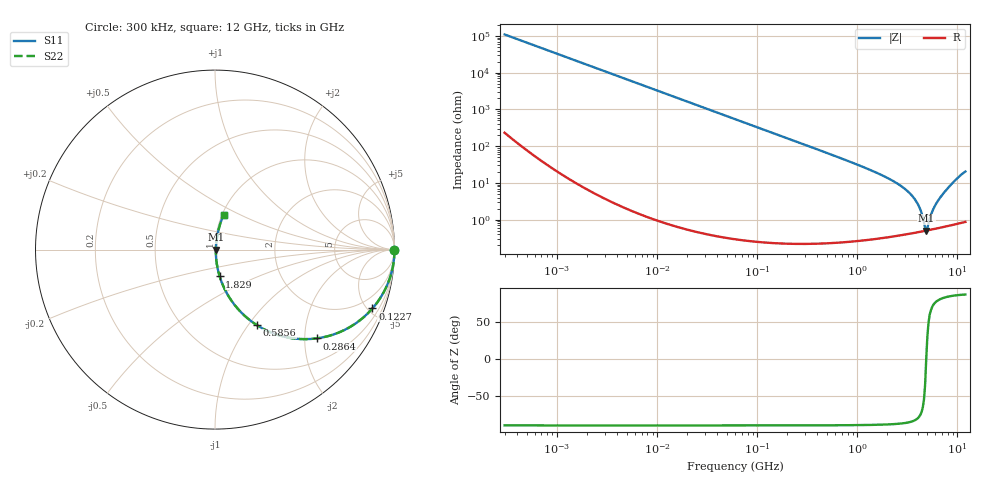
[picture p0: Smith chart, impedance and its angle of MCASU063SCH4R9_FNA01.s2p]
! MCASU063SCH4R9_FNA01  S-PARAMETER MODEL  ( General Type )
! Model Generated by TAIYO YUDEN Corporation (http://www.ty-top.com)
! Version 1.0
! TAIYO YUDEN Control No. 130801
! Copyright(c) 2013 TAIYO YUDEN CO.,LTD. All Rights Reserved.
! Product Description (link to TY-COMPAS)
! https://ds.yuden.co.jp/TYCOMPAS/or/detail?pn=MCASU063SCH4R9CFNA01&u=M
! Products Name : Multilayer Ceramic Capacitors
! Characteristics :
!  Capacitance : 4.9 pF , Rated Voltage : 50V , TCC : CH / C0H
!  Case Size : 0.6 x 0.3 / 0.024 x 0.012 [mm/inch] , Thickness : 0.3 / 0.012 [mm/inch]
!  (Conditions: Temperature = 25 degC , DC Bias Current/Voltage = 0A / 0V)
! External Node Assignments :
!  1  o---| |---o  2
! GND o---------o GND
! Frequency Range : 0.3MHz  -  12000MHz  [ 401 STEP ]
# MHz S RI R 50
! Freq[MHz].  S11 Real  S11 Imag  S21 Real  S21 Imag  S12 Real  S12 Imag  S22 Real  S22 Imag
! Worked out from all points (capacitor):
!   401 points, 300 kHz to 12 GHz, reference 50 ohm
!   read as one part in series: C = 4.85 pF near 316.3 kHz
!   lowest |Z| = 503 mohm at 4.875 GHz (marker M1)
!   series resonance near 4.876 GHz, so ESL is about 220 pH
!   S11 on the Smith chart (normalised r, x): 300 kHz: open; 122.7 MHz: 1.00, -5.35; 286.4 MHz: 1.00, -2.28; 585.6 MHz: 1.00, -1.10; 1.829 GHz: 1.01, -0.31; 12 GHz: 1.02, +0.41
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0.3  1 -0.000914  2.77e-06 0.000914  2.77e-06 0.000914  1 -0.000914
1.769972  1 -0.00539  3.14e-05 0.00539  3.14e-05 0.00539  1 -0.00539
10.44266  0.999 -0.0318  0.00102 0.0318  0.00102 0.0318  0.999 -0.0318
60  0.9676 -0.1769  0.0324 0.1769  0.0324 0.1769  0.9676 -0.1769
122.6847  0.877 -0.328  0.123 0.328  0.123 0.328  0.877 -0.328
182.544  0.7629 -0.4247  0.2371 0.4247  0.2371 0.4247  0.7629 -0.4247
286.3882  0.5658 -0.4947  0.4342 0.4947  0.4342 0.4947  0.5658 -0.4947
353.9943  0.4597 -0.4972  0.5403 0.4972  0.5403 0.4972  0.4597 -0.4972
585.5907  0.2347 -0.4217  0.7653 0.4217  0.7653 0.4217  0.2347 -0.4217
968.706  0.0976 -0.2929  0.9024 0.2929  0.9024 0.2929  0.0976 -0.2929
1829.429  0.0262 -0.1496  0.9738 0.1496  0.9738 0.1496  0.0262 -0.1496
2088.533  0.0194 -0.1254  0.9806 0.1254  0.9806 0.1254  0.0194 -0.1254
2870.14  0.00933 -0.0737  0.9907 0.0737  0.9907 0.0737  0.00933 -0.0737
3642.919  0.00587 -0.0394  0.9941 0.0394  0.9941 0.0394  0.00587 -0.0394
4158.869  0.00506 -0.0213  0.9949 0.0213  0.9949 0.0213  0.00506 -0.0213
4623.766  0.00492 -0.00706  0.9951 0.00706  0.9951 0.00706  0.00492 -0.00706
4875.354  0.00501 -6.78e-06  0.995 6.78e-06  0.995 6.78e-06  0.00501 -6.78e-06
5140.631  0.00519 0.00601  0.9948 -0.00601  0.9948 -0.00601  0.00519 0.00601
5868.704  0.006 0.0211  0.994 -0.0211  0.994 -0.0211  0.006 0.0211
6699.894  0.00749 0.0385  0.9925 -0.0385  0.9925 -0.0385  0.00749 0.0385
9207.246  0.0186 0.1054  0.9814 -0.1054  0.9814 -0.1054  0.0186 0.1054
12000  0.0475 0.1923  0.9525 -0.1923  0.9525 -0.1923  0.0475 0.1923
